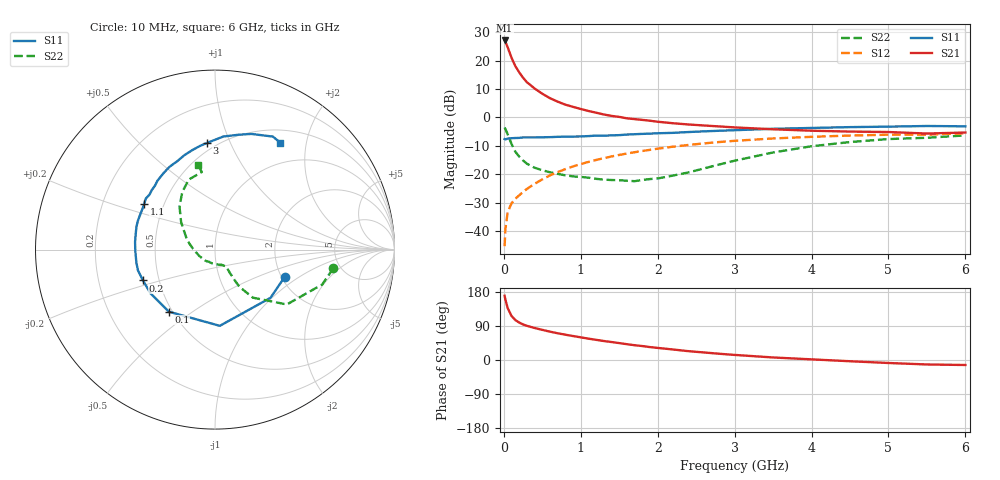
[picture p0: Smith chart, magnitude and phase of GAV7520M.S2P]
! Infineon Technologies  Discrete & RF Semiconductors
! BF775
! Si NPN RF Bipolar Junction Transistor in SOT23
! VCE = 0.75 V  IC = 20 mA
! Common Emitter S-Parameters:  May  1996
# GHz  S  MA  R  50
!  f  S11  S21  S12  S22
! GHz  MAG  ANG  MAG  ANG  MAG  ANG  MAG  ANG
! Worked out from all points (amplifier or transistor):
!   36 points, 10 MHz to 6 GHz, reference 50 ohm
!   highest |S21| = 27.1 dB at 10 MHz (marker M1)
!   |S21| within 3 dB of that: start of sweep to 57.99 MHz
!   unconditionally stable (mu >= 1): start of sweep to 29.33 MHz; 82.42 MHz to end of sweep
!   at 250 MHz: K = 1.65, MAG = 15.4 dB, |S12| = -26.3 dB
!   at 1.4 GHz: K = 1.83, MAG = 1.9 dB, |S12| = -13.7 dB
!   at 6 GHz: K = 1.17, MAG = -2.3 dB, |S12| = -5.6 dB
!   S11 on the Smith chart (normalised r, x): 10 MHz: 2.07, -0.77; 100 MHz: 0.48, -0.41; 200 MHz: 0.41, -0.17; 1.1 GHz: 0.39, +0.25; 3 GHz: 0.45, +0.82; 6 GHz: 0.67, +1.57
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0.01  0.4168 -21.6  22.73 169.5  0.0054 78.3  0.6671 -9.0
0.02  0.4096 -41.0  21.6 159.5  0.0107 72.3  0.6282 -18.0
0.05  0.4256 -86.4  17.22 136.9  0.0216 59.1  0.5035 -37.4
0.1  0.4309 -126.6  11.26 116.2  0.0307 52.9  0.3414 -51.7
0.15  0.4343 -146.0  7.989 105.2  0.0371 52.9  0.2484 -56.7
0.2  0.4365 -156.8  6.233 98.8  0.0425 55.3  0.2041 -57.3
0.25  0.4446 -164.9  4.999 93.8  0.0486 57.4  0.1746 -57.3
0.3  0.444 -170.5  4.18 90.2  0.055 59.8  0.1532 -57.5
0.4  0.4442 -179.2  3.237 84.5  0.0679 62.3  0.1301 -56.9
0.5  0.4475 174.4  2.617 79.5  0.0811 63.6  0.1174 -56.5
0.6  0.4501 169.0  2.184 74.8  0.0953 64.4  0.1082 -58.4
0.7  0.4559 163.7  1.898 70.5  0.1089 64.3  0.1014 -61.4
0.8  0.4584 159.9  1.68 66.8  0.1231 63.6  0.0956 -64.3
1.1  0.4696 147.2  1.301 56.3  0.1646 61.2  0.0869 -76.6
1.3  0.4764 139.9  1.128 50.1  0.192 58.9  0.0804 -87.7
1.6  0.4998 130.0  0.965 41.7  0.2316 54.7  0.0767 -110.6
2.2  0.5356 113.1  0.791 27.7  0.3056 45.5  0.0946 -158.2
3  0.5962 94.2  0.668 13.4  0.3877 32.6  0.1731 157.4
3.5  0.6317 85.8  0.619 6.7  0.4263 24.8  0.2415 141.3
4.5  0.6758 72.5  0.564 -3.3  0.4801 10.6  0.3688 119.6
5.5  0.7075 62.9  0.521 -11.8  0.4963 -2.3  0.4386 99.6
6  0.6982 58.7  0.543 -13.2  0.5274 -6.0  0.4828 101.6
